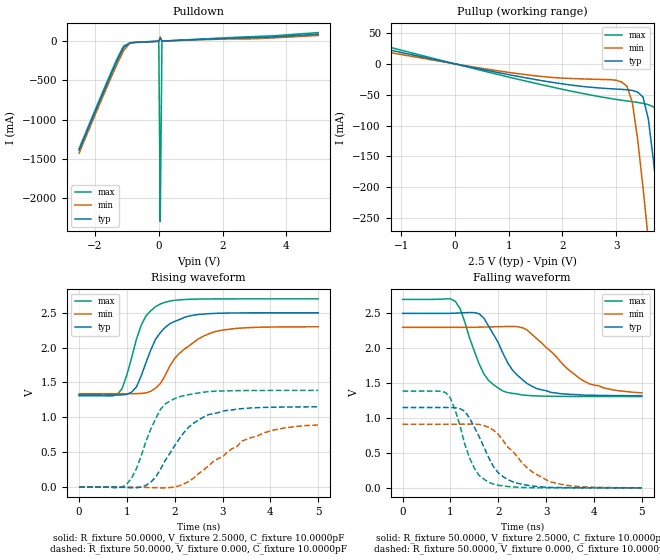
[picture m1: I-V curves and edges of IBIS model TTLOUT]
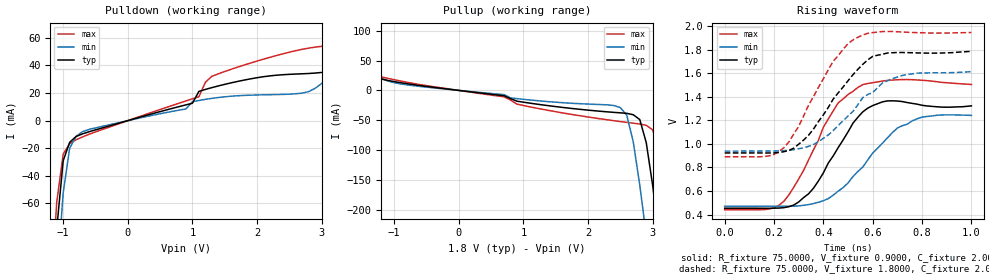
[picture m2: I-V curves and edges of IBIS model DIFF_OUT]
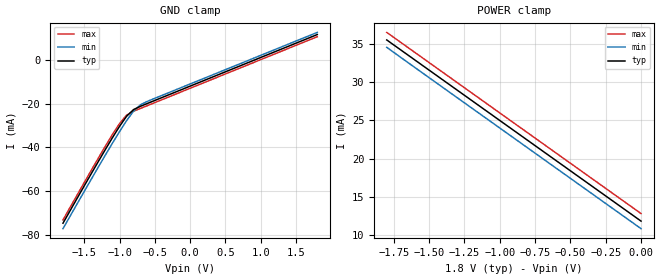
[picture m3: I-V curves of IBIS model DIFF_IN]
[IBIS ver]   2.1
[File name]   warp217_25_75.ibs
[File Rev]   1.0
[Date]   January 10, 2000
[Source]   Motorola, data from spice models.
[Notes]   This model represents the MC92600 WarpLink Quad Gigabit
   transceiver using 2.5 V TTL I/O power driving 75 ohm media in
   a 217 PBGA
[Disclaimer]   This is a preliminary model for review purposes only.
[Copyright]   Copyright 2000 Motorola Inc.
|   Component MC92600
[Component]   MC92600
[Manufacturer]   Motorola Inc.
[Package]
| variable   typ   min   max
R_pkg   0.1500   NA   NA
L_pkg   6.8000nH   NA   NA
C_pkg   1.7000pF   NA   NA
[Pin]  signal_name   model_name   R_pin   L_pin   C_pin
B3   recv_d_5   TTLOUT
C2   recv_d_4   TTLOUT
B1   recv_d_3   TTLOUT
C1   recv_d_2   TTLOUT
C3   recv_d_1   TTLOUT
D2   recv_d_0   TTLOUT
D1   recv_c_0   TTLOUT
D3   recv_c_1   TTLOUT
E2   recv_c_2   TTLOUT
E3   recv_c_3   TTLOUT
F2   recv_c_4   TTLOUT
F1   recv_c_5   TTLOUT
G2   recv_c_6   TTLOUT
F3   recv_c_7   TTLOUT
G1   recv_c_k   TTLOUT
H2   recv_c_9   TTLOUT
H1   recv_c_rclk   TTLOUT
J1   recv_c_idle   TTLOUT
H3   recv_c_err   TTLOUT
J2   recv_b_err   TTLOUT
K1   recv_b_idle   TTLOUT
K2   recv_b_rclk   TTLOUT
J3   recv_b_9   TTLOUT
L1   recv_b_k   TTLOUT
L2   recv_b_7   TTLOUT
M1   recv_b_6   TTLOUT
L3   recv_b_5   TTLOUT
M2   recv_b_4   TTLOUT
N1   recv_b_3   TTLOUT
M3   recv_b_2   TTLOUT
P1   recv_b_1   TTLOUT
P2   recv_b_0   TTLOUT
N3   recv_a_0   TTLOUT
R1   recv_a_1   TTLOUT
T1   recv_a_2   TTLOUT
P3   recv_a_3   TTLOUT
N4   recv_a_4   TTLOUT
R3   recv_a_5   TTLOUT
T2   recv_a_6   TTLOUT
T3   recv_a_7   TTLOUT
U3   recv_a_k   TTLOUT
T4   recv_a_9   TTLOUT
U4   recv_a_rclk   TTLOUT
R4   recv_a_idle   TTLOUT
R5   recv_a_err   TTLOUT
T5   xmit_b_idle_b   TTLIN
U5   xmit_b_k   TTLIN
T6   xmit_b_7   TTLIN
R6   xmit_b_6   TTLIN
U6   xmit_b_5   TTLIN
T7   xmit_b_4   TTLIN
U7   xmit_b_3   TTLIN
R7   xmit_b_2   TTLIN
T8   xmit_b_1   TTLIN
R8   xmit_b_0   TTLIN
U8   xmit_a_0   TTLIN
U10   xmit_a_1   TTLIN
T10   xmit_a_2   TTLIN
R10   xmit_a_3   TTLIN
U11   xmit_a_4   TTLIN
T11   xmit_a_5   TTLIN
R11   xmit_a_6   TTLIN
T12   xmit_a_7   TTLIN
T13   xmit_a_k   TTLIN
U13   tst_1   TTLIN
R12   wse_gen   TTLIN
T14   xmit_a_idle_b   TTLIN
U14   tst_0   TTLIN
U15   bsync_1   TTLIN
R13   bsync_0   TTLIN
R14   lbe   TTLIN
P13   lboe   TTLIN
T15   tbie   TTLIN
R16   media   TTLIN
P17   rlk_a_n   DIFF_IN
N17   rlk_a_p   DIFF_IN
N15   xlk_a_n   DIFF_OUT
M15   xlk_a_p   DIFF_OUT
M14   xlk_b_p   DIFF_OUT
L14   xlk_b_n   DIFF_OUT
L17   rlk_b_p   DIFF_IN
K17   rlk_b_n   DIFF_IN
K15   pll_tpa   NC
H17   rlk_c_n   DIFF_IN
G17   rlk_c_p   DIFF_IN
H14   xlk_c_n   DIFF_OUT
G14   xlk_c_p   DIFF_OUT
G15   xlk_d_p   DIFF_OUT
F15   xlk_d_n   DIFF_OUT
E17   rlk_d_p   DIFF_IN
D17   rlk_d_n   DIFF_IN
C16   repe   TTLIN
E14   rcce   TTLIN
C15   adie   TTLIN
B16   wse   TTLIN
B15   hse   TTLIN
C14   ddre   TTLIN
A15   ref_clk   TTLIN
B14   reset_b   TTLIN
A14   stndby   TTLIN
D13   xmit_d_idle_b   TTLIN
B13   xmit_d_k   TTLIN
A13   xmit_d_7   TTLIN
C13   xmit_d_6   TTLIN
B12   xmit_d_5   TTLIN
A12   xmit_d_4   TTLIN
B11   xmit_d_3   TTLIN
A11   xmit_d_2   TTLIN
C11   xmit_d_1   TTLIN
C10   xmit_d_0   TTLIN
B10   xmit_c_0   TTLIN
A10   xmit_c_1   TTLIN
C8   xmit_c_2   TTLIN
B8   xmit_c_3   TTLIN
A8   xmit_c_4   TTLIN
A7   xmit_c_5   TTLIN
B7   xmit_c_6   TTLIN
C7   xmit_c_7   TTLIN
A6   xmit_c_k   TTLIN
B6   xmit_c_idle_b   TTLIN
C6   recv_d_err   TTLOUT
B5   recv_d_idle   TTLOUT
A4   recv_d_rclk   TTLOUT
C5   recv_d_9   TTLOUT
C4   recv_d_k   TTLOUT
B4   recv_d_7   TTLOUT
A3   recv_d_6   TTLOUT
A1   GND   GND
H9   GND   GND
P4   GND   GND
A17   GND   GND
H10   GND   GND
P6   GND   GND
B2   GND   GND
J8   GND   GND
P8   GND   GND
D4   GND   GND
J9   GND   GND
P10   GND   GND
D6   GND   GND
J10   GND   GND
P12   GND   GND
D8   GND   GND
K4   GND   GND
P14   GND   GND
D10   GND   GND
K8   GND   GND
R15   GND   GND
D12   GND   GND
K9   GND   GND
T16   GND   GND
F4   GND   GND
K10   GND   GND
U1   GND   GND
H4   GND   GND
M4   GND   GND
U17   GND   GND
H8   GND   GND
F17   GND   GND
H15   GND   GND
J14   GND   GND
L15   GND   GND
M17   GND   GND
J16   GND   GND
C17   GND   GND
D15   GND   GND
E15   GND   GND
F14   GND   GND
J17   GND   GND
N14   GND   GND
P15   GND   GND
R17   GND   GND
T17   GND   GND
K16   GND   GND
F16   VDD18   POWER
G16   VDD18   POWER
J15   VDD18   POWER
M16   VDD18   POWER
N16   VDD18   POWER
B17   VDD18   POWER
D14   VDD18   POWER
D16   VDD18   POWER
E16   VDD18   POWER
H16   VDD18   POWER
K14   VDD18   POWER
L16   VDD18   POWER
P16   VDD33   POWER
A5   VDD33   POWER
C12   VDD33   POWER
E1   VDD33   POWER
E4   VDD33   POWER
G3   VDD33   POWER
K3   VDD33   POWER
N2   VDD33   POWER
P5   VDD33   POWER
R2   VDD33   POWER
U12   VDD33   POWER
A2   VDD18   POWER
A9   VDD18   POWER
A16   VDD18   POWER
B9   VDD18   POWER
C9   VDD18   POWER
D5   VDD18   POWER
D7   VDD18   POWER
D9   VDD18   POWER
D11   VDD18   POWER
G4   VDD18   POWER
J4   VDD18   POWER
L4   VDD18   POWER
P7   VDD18   POWER
P9   VDD18   POWER
P11   VDD18   POWER
R9   VDD18   POWER
T9   VDD18   POWER
U2   VDD18   POWER
U9   VDD18   POWER
U16   VDD18   POWER
[Diff Pin]  inv_pin  vdiff   tdelay_typ  tdelay_min  tdelay_max
N17   P17   0.2000V  NA   NA   NA
M15   N15   NA   NA   NA   NA
L17   K17   0.2000V  NA   NA   NA
M14   L14   NA   NA   NA   NA
G17   H17   0.2000V  NA   NA   NA
G14   H14   NA   NA   NA   NA
E17   D17   0.2000V  NA   NA   NA
G15   F15   NA   NA   NA   NA
| Models and submodels in the file (4): TTLOUT (Output), DIFF_OUT (Output), DIFF_IN (Input), TTLIN (Input)
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|   Model TTLOUT
[Model]   TTLOUT
Model_type   Output
Vmeas =   1.5000V
Cref =  10.0000pF
Rref =   0.5000k
Vref =  0.000V
C_comp   3.9200pF   NA   NA
[Temperature Range]   40.0000   0.1050k   0.000
[Pullup Reference]   2.5000V   2.3000V   2.7000V
[Pulldown Reference]   0.000V   0.000V   0.000V
[POWER Clamp Reference]   2.5000V   2.3000V   2.7000V
[GND Clamp Reference]   0.000V   0.000V   0.000V
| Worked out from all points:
|   slope of the pulldown table from 0 to 0.375 V, typ, clamps not added: 54.1 ohm
|   slope of the pullup table from 0 to 0.375 V, typ, clamps not added: 55.7 ohm
|   rising waveform, R_fixture 50.0000, V_fixture 2.5000, C_fixture 10.0000pF: 20-80 % time 489ps typ, 719ps min, 386ps max; typ from 1.32 V to 2.5 V
|   rising waveform, R_fixture 50.0000, V_fixture 0.000, C_fixture 10.0000pF: 20-80 % time 723ps typ, 1.14ns min, 490ps max; typ from 0 V to 1.15 V
|   falling waveform, R_fixture 50.0000, V_fixture 2.5000, C_fixture 10.0000pF: 20-80 % time 651ps typ, 898ps min, 470ps max; typ from 2.5 V to 1.32 V
|   falling waveform, R_fixture 50.0000, V_fixture 0.000, C_fixture 10.0000pF: 20-80 % time 522ps typ, 780ps min, 403ps max; typ from 1.15 V to 0 V
[Pulldown]
| voltage   I(typ)   I(min)   I(max)
-2.5V     -1.391A    -1.429A    -1.371A
-1.5V     -424.9mA   -467.2mA   -401mA
-1.3V     -241.6mA   -284.6mA   -217.1mA
-1.1V     -79.34mA   -117.9mA   -59.55mA
-900mV    -19.22mA   -22.77mA   -20.24mA
0V        -7.924nA   -193.5nA   -49.23nA
31.6mV    25.95mA    37.78mA    -1.5A
46.6mV    39.35mA    55.66mA    -2.3A
100mV     1.862mA    1.543mA    2.187mA
3.1V      47.93mA    33.19mA    61.7mA
5V        90.19mA    73.57mA    110.6mA
[Pullup]
| voltage   I(typ)   I(min)   I(max)
-2.5V     46.59mA    39.35mA    55.66mA
1V        -17.46mA   -13.77mA   -21.39mA
3.1V      -41.29mA   -29.36mA   -58.88mA
3.2V      -41.93mA   -36.15mA   -60.09mA
3.3V      -42.99mA   -61.92mA   -61.24mA
3.4V      -45.79mA   -122mA     -62.49mA
3.5V      -53.73mA   -200.4mA   -64.06mA
3.6V      -89.85mA   -286.4mA   -66.03mA
3.8V      -245mA     -468.3mA   -85.03mA
4V        -426.8mA   -656.4mA   -223mA
4.2V      -615.6mA   -847.6mA   -404mA
5V        -1.392A    -1.626A    -1.175A
[Ramp]
| variable   typ   min   max
dV/dt_r   0.6917/0.5170n   0.5461/0.8775n   0.8331/0.3448n
dV/dt_f   0.7089/0.3850n   0.5735/0.6401n   0.8363/0.2560n
R_load = 50.0000
[Rising Waveform]
R_fixture = 50.0000
V_fixture = 2.5000
V_fixture_min = 2.3000
V_fixture_max = 2.7000
C_fixture = 10.0000pF
R_dut = 0.1500
L_dut = 6.8000nH
C_dut = 1.7000pF
| time   V(typ)   V(min)   V(max)
0s        1.32V      1.339V     1.308V
800ps     1.32V      1.339V     1.328V
900ps     1.322V     1.339V     1.412V
1.2ns     1.436V     1.34V      2.121V
1.4ns     1.786V     1.351V     2.456V
1.6ns     2.121V     1.419V     2.588V
1.7ns     2.215V     1.484V     2.626V
2.1ns     2.403V     1.918V     2.685V
2.8ns     2.49V      2.221V     2.699V
5ns       2.5V       2.299V     2.7V
[Rising Waveform]
R_fixture = 50.0000
V_fixture = 0.000
V_fixture_min = 0.000
V_fixture_max = 0.000
C_fixture = 10.0000pF
R_dut = 0.1500
L_dut = 6.8000nH
C_dut = 1.7000pF
| time   V(typ)   V(min)   V(max)
0s        208.3nV    5.446uV    1.175uV
1ns       -7.456mV   294.8uV    44.06mV
1.2ns     -11.46mV   -1.124mV   263.7mV
1.5ns     70.48mV    -7.301mV   831.3mV
1.7ns     250.7mV    -11.33mV   1.112V
2ns       595.2mV    1.827mV    1.269V
2.3ns     862.8mV    83.08mV    1.326V
2.7ns     1.037V     299.9mV    1.369V
3.6ns     1.136V     710.9mV    1.385V
5ns       1.151V     891.4mV    1.386V
[Falling Waveform]
R_fixture = 50.0000
V_fixture = 2.5000
V_fixture_min = 2.3000
V_fixture_max = 2.7000
C_fixture = 10.0000pF
R_dut = 0.1500
L_dut = 6.8000nH
C_dut = 1.7000pF
| time   V(typ)   V(min)   V(max)
0s        2.5V       2.3V       2.7V
1.1ns     2.503V     2.3V       2.675V
1.2ns     2.506V     2.3V       2.569V
1.6ns     2.495V     2.302V     1.776V
1.8ns     2.315V     2.306V     1.536V
2.1ns     1.924V     2.31V      1.386V
2.3ns     1.685V     2.313V     1.354V
2.8ns     1.423V     2.14V      1.318V
3.8ns     1.328V     1.526V     1.309V
5ns       1.321V     1.361V     1.308V
[Falling Waveform]
R_fixture = 50.0000
V_fixture = 0.000
V_fixture_min = 0.000
V_fixture_max = 0.000
C_fixture = 10.0000pF
R_dut = 0.1500
L_dut = 6.8000nH
C_dut = 1.7000pF
| time   V(typ)   V(min)   V(max)
0s        1.151V     911.8mV    1.386V
900ps     1.152V     911.8mV    1.365V
1.1ns     1.148V     911.8mV    1.112V
1.3ns     1.097V     912.3mV    623.4mV
1.5ns     869.9mV    912.6mV    281.8mV
1.8ns     432.4mV    867.6mV    78.49mV
2.2ns     118.4mV    582.7mV    19.15mV
2.7ns     26.79mV    232.5mV    2.613mV
3.1ns     6.501mV    85.62mV    630.1uV
5ns       32.56uV    760.5uV    2.211uV
|   Model DIFF_OUT
[Model]   DIFF_OUT
Model_type   Output
Vmeas =   1.5000V
Cref =   2.0000pF
Rref =   0.5000k
Vref =   0.9000V
C_comp   3.1000pF   NA   NA
[Temperature Range]   40.0000   0.1050k   0.000
[Pullup Reference]   1.8000V   1.6500V   1.9500V
[Pulldown Reference]   0.000V   0.000V   0.000V
[POWER Clamp Reference]   1.8000V   1.6500V   1.9500V
[GND Clamp Reference]   0.000V   0.000V   0.000V
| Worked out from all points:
|   slope of the pulldown table from 0 to 0.27 V, typ, clamps not added: 75.5 ohm
|   slope of the pullup table from 0 to 0.27 V, typ, clamps not added: 77.3 ohm
|   rising waveform, R_fixture 75.0000, V_fixture 0.9000, C_fixture 2.0000pF: 20-80 % time 151ps typ, 198ps min, 157ps max; typ from 0.454 V to 1.32 V
|   rising waveform, R_fixture 75.0000, V_fixture 1.8000, C_fixture 2.0000pF: 20-80 % time 183ps typ, 202ps min, 169ps max; typ from 0.923 V to 1.78 V
[Pulldown]
| voltage   I(typ)   I(min)   I(max)
-1.8V     -710.2mA   -751mA     -687.5mA
-1.2V     -155.1mA   -197.5mA   -131.5mA
-1.1V     -78.49mA   -117.2mA   -59.17mA
-1V       -29.06mA   -52.31mA   -24.26mA
-900mV    -15.71mA   -19.96mA   -16.69mA
-800mV    -11.49mA   -11.41mA   -13.85mA
1V        12.61mA    13.72mA    15.81mA
1.3V      23.92mA    16.12mA    32.11mA
2.8V      34.17mA    21.06mA    52.57mA
3.2V      36.29mA    37.97mA    54.77mA
3.4V      40.79mA    82.89mA    56.11mA
3.6V      57.28mA    198.6mA    58.1mA
[Pullup]
| voltage   I(typ)   I(min)   I(max)
-1.8V     54.64mA    105.3mA    50.62mA
-1.6V     36.62mA    42.56mA    39.21mA
-1.4V     27.4mA     27.38mA    29.58mA
2.4V      -36.74mA   -25.27mA   -50.71mA
2.6V      -38.39mA   -41.74mA   -53.55mA
2.7V      -40.76mA   -86.81mA   -54.91mA
2.9V      -87.34mA   -242.1mA   -58.38mA
3V        -159.5mA   -330.5mA   -66.06mA
3.1V      -244.2mA   -421.7mA   -105.1mA
3.2V      -333.9mA   -514.6mA   -179.6mA
3.3V      -426.3mA   -608.8mA   -266mA
3.6V      -711.1mA   -895.5mA   -545.1mA
[Ramp]
| variable   typ   min   max
dV/dt_r   0.5403/0.1253n   0.4234/0.2140n   0.6550/79.1927p
dV/dt_f   0.4180/77.5717p   0.4013/0.1925n   0.5154/52.6923p
R_load = 50.0000
[Rising Waveform]
R_fixture = 75.0000
V_fixture = 0.9000
V_fixture_min = 0.8250
V_fixture_max = 0.9750
C_fixture = 2.0000pF
R_dut = 0.1500
L_dut = 6.8000nH
C_dut = 1.7000pF
| time   V(typ)   V(min)   V(max)
0s        454.4mV    471.3mV    441.4mV
200ps     454.2mV    470.7mV    457.8mV
240ps     458.9mV    470.3mV    513.1mV
300ps     507.5mV    473.9mV    702.4mV
360ps     624.3mV    493.5mV    950.6mV
460ps     968.5mV    599.3mV    1.348V
560ps     1.272V     804.2mV    1.503V
660ps     1.365V     1.052V     1.538V
760ps     1.344V     1.196V     1.545V
1ns       1.323V     1.241V     1.504V
[Rising Waveform]
R_fixture = 75.0000
V_fixture = 1.8000
V_fixture_min = 1.6500
V_fixture_max = 1.9500
C_fixture = 2.0000pF
R_dut = 0.1500
L_dut = 6.8000nH
C_dut = 1.7000pF
| time   V(typ)   V(min)   V(max)
0s        923.2mV    938.9mV    891mV
180ps     922.8mV    939.2mV    898.1mV
240ps     933.8mV    942.8mV    967.9mV
300ps     997.5mV    959mV      1.149V
340ps     1.074V     979mV      1.329V
440ps     1.381V     1.113V     1.702V
540ps     1.633V     1.333V     1.905V
600ps     1.742V     1.435V     1.944V
720ps     1.775V     1.58V      1.949V
1ns       1.785V     1.613V     1.945V
|   Model DIFF_IN
[Model]   DIFF_IN
Model_type   Input
C_comp   1.0000pF   NA   NA
[Temperature Range]   40.0000   0.1050k   0.000
[Pullup Reference]   1.8000V   1.6500V   1.9500V
[Pulldown Reference]   0.000V   0.000V   0.000V
[POWER Clamp Reference]   1.8000V   1.6500V   1.9500V
[GND Clamp Reference]   0.000V   0.000V   0.000V
[GND_clamp]
| voltage   I(typ)   I(min)   I(max)
-1.8V     -74.78mA   -77.29mA   -73.27mA
-1.3V     -46.45mA   -49.01mA   -44.91mA
-1.1V     -35.51mA   -38.04mA   -34.04mA
-1V       -30.33mA   -32.74mA   -29.03mA
-900mV    -25.68mA   -27.7mA    -25.16mA
-800mV    -22.58mA   -23.29mA   -23.37mA
-700mV    -21.06mA   -20.34mA   -22.04mA
1.8V      11.84mA    12.83mA    10.86mA
[POWER_clamp]
| voltage   I(typ)   I(min)   I(max)
-1.8V     35.53mA    34.56mA    36.51mA
-1.7V     34.21mA    33.23mA    35.2mA
-1.5V     31.58mA    30.59mA    32.57mA
0V        11.84mA    10.86mA    12.83mA
